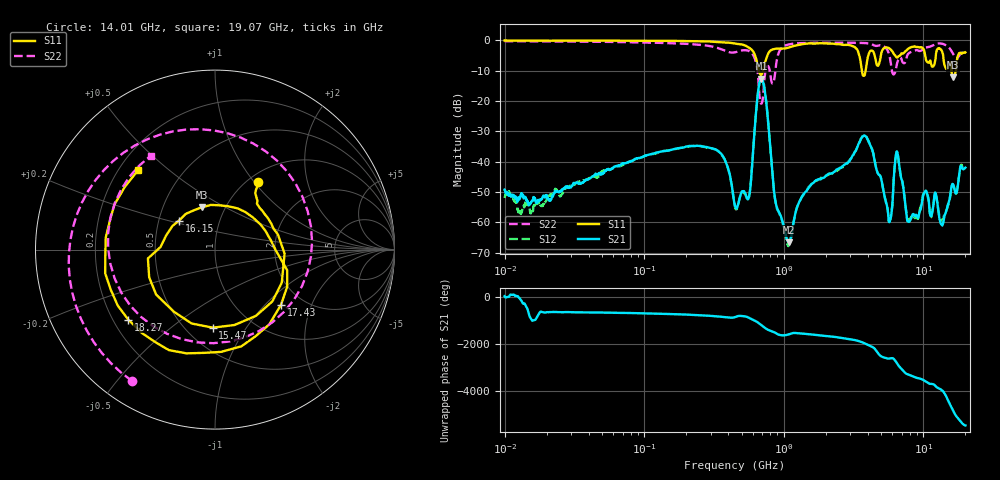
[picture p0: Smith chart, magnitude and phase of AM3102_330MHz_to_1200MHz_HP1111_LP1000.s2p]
! Date/Time: Tue, Sep 11, 2018 5:24 PM
! Network Analyzer: Agilent Technologies E8362B Rev: A.07.50.63
! Sweep from 0.010 to 20.000 GHz, 1601 Points, Sweep Type: LOG
! Power Supply: 4.949 V, 0.001 A
# Hz S DB R 50
!freq MagS11 AngS11 MagS21 AngS21 MagS12 AngS12 MagS22 AngS22
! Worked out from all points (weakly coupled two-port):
!   1601 points, 10 MHz to 20 GHz, reference 50 ohm
!   highest |S21| = -12.60 dB at 692.3 MHz (marker M1); lowest = -66.6 dB at 1.082 GHz (marker M2)
!   lowest |S11| = -12.2 dB at 16.38 GHz (marker M3), VSWR 1.66, Z = 38.9 + j19.5 ohm
!   |S11| at or under -10 dB: 663.7 MHz to 709.9 MHz (46.19 MHz wide, 6.73 % of centre); 3.624 GHz to 3.854 GHz (229.8 MHz wide, 6.15 % of centre); 15.91 GHz to 17.11 GHz (1.197 GHz wide, 7.25 % of centre)
!   |S22| runs from -20.9 to -0.3 dB; largest |S21 - S12| = 0.0057
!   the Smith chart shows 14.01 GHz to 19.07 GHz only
!   S11 on the Smith chart (normalised r, x): 14.01 GHz: 1.11, +1.05; 15.47 GHz: 0.67, -0.72; 16.15 GHz: 0.64, +0.22; 17.43 GHz: 1.56, -1.24; 18.27 GHz: 0.26, -0.33; 19.07 GHz: 0.28, +0.40
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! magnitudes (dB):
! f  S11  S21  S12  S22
! 10 MHz  0.0  -49.2  -52.0  -0.3
! 35.55 MHz  -0.1  -47.2  -46.5  -0.4
! 126.4 MHz  -0.2  -36.8  -37.0  -0.8
! 336.3 MHz  -0.6  -36.4  -36.4  -2.5
! 447.2 MHz  -1.0  -54.5  -54.9  -3.9
! 564.4 MHz  -2.4  -51.5  -51.4  -3.5
! 692.3 MHz  -11.3  -12.6  -12.6  -20.9
! 873.8 MHz  -2.7  -53.3  -53.7  -9.2
! 1.082 GHz  -2.3  -66.6  -67.7  -1.3
! 1.59 GHz  -1.0  -47.3  -47.3  -0.8
! 3.811 GHz  -11.2  -31.4  -31.3  -0.8
! 5.652 GHz  -2.5  -59.6  -59.4  -4.3
! 6.487 GHz  -5.6  -36.7  -36.9  -7.4
! 7.845 GHz  -2.7  -59.8  -59.1  -4.3
! 14.01 GHz  -7.0  -59.3  -58.1  -1.3
! 15.47 GHz  -7.2  -51.9  -52.3  -2.7
! 16.15 GHz  -11.8  -47.4  -47.6  -4.0
! 16.38 GHz  -12.2  -47.6  -47.7  -4.5
! 17.43 GHz  -6.4  -49.6  -49.5  -5.7
! 18.27 GHz  -4.1  -42.5  -42.4  -4.7
! 19.07 GHz  -4.2  -42.4  -41.8  -4.0
! 20 GHz  -4.0  -42.0  -42.4  -4.0
